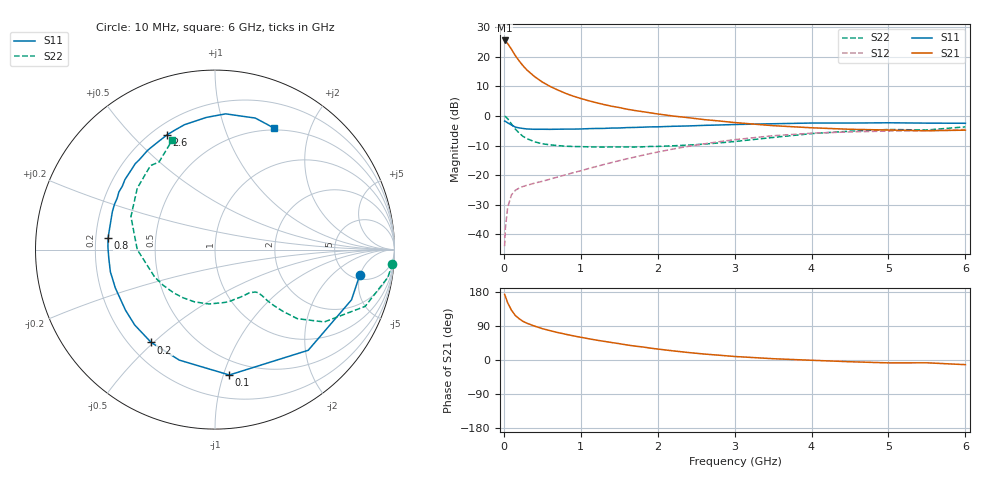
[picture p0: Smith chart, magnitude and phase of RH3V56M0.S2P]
! SIEMENS Small Signal Semiconductors
! BFR106
! Si NPN RF Bipolar Junction Transistor in SOT23
! VCE = 3.5 V  IC = 6 mA
! Common Emitter S-Parameters:  August  1996
# GHz  S  MA  R  50
!  f  S11  S21  S12  S22
! GHz  MAG  ANG  MAG  ANG  MAG  ANG  MAG  ANG
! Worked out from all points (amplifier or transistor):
!   36 points, 10 MHz to 6 GHz, reference 50 ohm
!   highest |S21| = 25.5 dB at 10 MHz (marker M1)
!   |S21| within 3 dB of that: start of sweep to 99.81 MHz
!   unconditionally stable (mu >= 1): 579.5 MHz to 2.038 GHz; 4.774 GHz to end of sweep
!   at 250 MHz: K = 0.56, MSG = 20.4 dB, |S12| = -23.8 dB
!   at 1.4 GHz: K = 1.13, MAG = 7.4 dB, |S12| = -15.8 dB
!   at 6 GHz: K = 1.02, MAG = -1.0 dB, |S12| = -4.6 dB
!   S11 on the Smith chart (normalised r, x): 10 MHz: 5.66, -4.93; 100 MHz: 0.38, -1.05; 200 MHz: 0.29, -0.49; 800 MHz: 0.25, +0.05; 2.6 GHz: 0.26, +0.63; 6 GHz: 0.48, +1.49
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0.01  0.8187 -10.1  18.86 173.1  0.0063 86.5  0.9911 -4.5
0.02  0.8104 -20.2  18.53 167.7  0.0126 79.2  0.9757 -9.1
0.05  0.7644 -47.2  16.67 150.8  0.0288 66.6  0.8944 -20.7
0.1  0.7031 -83.5  13.34 131.2  0.0465 53.3  0.7304 -33.5
0.15  0.6471 -107.9  10.42 117.3  0.0555 44.5  0.5985 -40.0
0.2  0.6277 -124.5  8.475 108.8  0.0605 41.5  0.5136 -42.2
0.25  0.6137 -136.8  7.029 101.8  0.0643 39.9  0.4504 -43.6
0.3  0.6022 -145.9  5.98 97.1  0.0673 40.6  0.4137 -44.2
0.4  0.595 -158.9  4.618 89.4  0.0732 41.9  0.3654 -44.4
0.5  0.5959 -168.0  3.74 82.8  0.0786 44.8  0.3388 -45.0
0.6  0.5937 -175.4  3.161 77.5  0.0855 47.3  0.3246 -46.7
0.8  0.5992 173.7  2.415 68.1  0.101 52.4  0.3079 -51.5
1.1  0.6097 159.7  1.811 56.2  0.1291 57.9  0.3005 -61.4
1.3  0.6156 152.3  1.56 49.3  0.1511 59.7  0.2977 -69.0
1.6  0.6354 142.2  1.302 39.7  0.1886 60.5  0.2989 -82.1
2.2  0.6686 124.1  0.996 24.1  0.2758 56.7  0.313 -111.8
2.6  0.6928 112.7  0.868 15.8  0.3371 51.2  0.3336 -133.9
3.5  0.7381 93.7  0.685 3.4  0.4633 35.2  0.4332 180.0
4.5  0.7583 78.6  0.595 -4.6  0.5374 16.4  0.5523 141.6
5  0.7665 73.0  0.578 -7.6  0.555 8.7  0.5901 127.5
5.5  0.7561 67.6  0.562 -7.4  0.5643 4.9  0.5791 122.6
6  0.7519 63.9  0.575 -12.3  0.5915 -2.9  0.6541 111.4
